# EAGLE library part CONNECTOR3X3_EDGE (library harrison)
3x3 edge connector
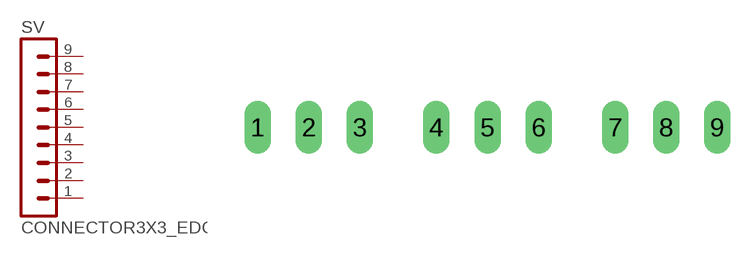
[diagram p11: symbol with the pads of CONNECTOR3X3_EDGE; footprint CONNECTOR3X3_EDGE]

Designator prefix SV

## CONNECTOR3X3_EDGE  [CONNECTOR3X3_EDGE]
1  1  pas
2  2  pas
3  3  pas
4  4  pas
5  5  pas
6  6  pas
7  7  pas
8  8  pas
9  9  pas

## Footprint CONNECTOR3X3_EDGE (pad centres in mm)
drill 0.813 long: 1 -11.43,0; 2 -8.89,0; 3 -6.35,0; 4 -2.54,0; 5 0,0; 6 2.54,0; 7 6.35,0; 8 8.89,0; 9 11.43,0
